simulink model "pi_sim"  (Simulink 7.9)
settings: Solver=FixedStepDiscrete  SolverMode=SingleTasking  StartTime=0.0  StopTime=500  FixedStep=1  RelTol=1e-3  AbsTol=1e-6
PreLoadFcn:
  | init_exercise
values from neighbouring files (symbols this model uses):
  w1 = 0.1    [init_exercise.m]
  w2 = 1.0    (= 1)    [init_exercise.m]
undefined symbols (not defined in the file or in its folder): DiscIntNeverNeededParam
libraries: labmvlib x1

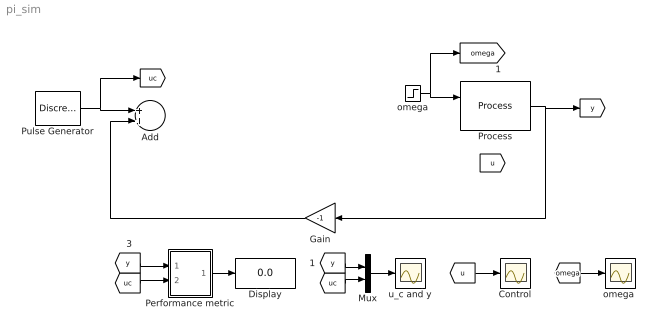
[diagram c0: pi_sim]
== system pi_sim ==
  Add : Sum
  Control : Scope
  Display : Display
  Gain : Gain  Gain=-1  SampleTime=1
  Mux : Mux  Inputs=2
  Performance metric : Subsystem
  Process : labmvlib/Process
  Pulse Generator : DiscretePulseGenerator  PulseType=Time based  Amplitude=5  Period=100  PulseWidth=50
  omega : Step  Time=250  Before=w1  After=w2  SampleTime=1
  "omega " : Scope
  u_c and y : Scope
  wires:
  omega/1 -> Process/1, [omega]
  ? -> Process/2, [u]
  Add/1 -> ?
  Gain/1 -> Add/2
  Mux/1 -> u_c and y/1
  Process/1 -> Gain/1, [y]
  Pulse Generator/1 -> Add/1, [uc]
  Performance metric/1(E) -> Display/1
  [uc] -> Mux/2
  [y] -> Mux/1
  [y] -> Performance metric/1(y)
  [uc] -> Performance metric/2(uc)
  [u] -> Control/1
  [omega] -> "omega "/1

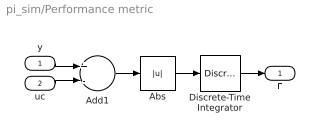
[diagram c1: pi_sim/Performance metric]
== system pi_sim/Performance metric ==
  y : Inport
  uc : Inport  Port=2
  Abs : Abs
  Add1 : Sum  Inputs=+-
  Discrete-Time Integrator : DiscreteIntegrator  ICPrevOutput=DiscIntNeverNeededParam  ICPrevScaledInput=DiscIntNeverNeededParam
  E : Outport
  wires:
  Abs/1 -> Discrete-Time Integrator/1
  Add1/1 -> Abs/1
  y/1 -> Add1/1
  Discrete-Time Integrator/1 -> E/1
  uc/1 -> Add1/2
